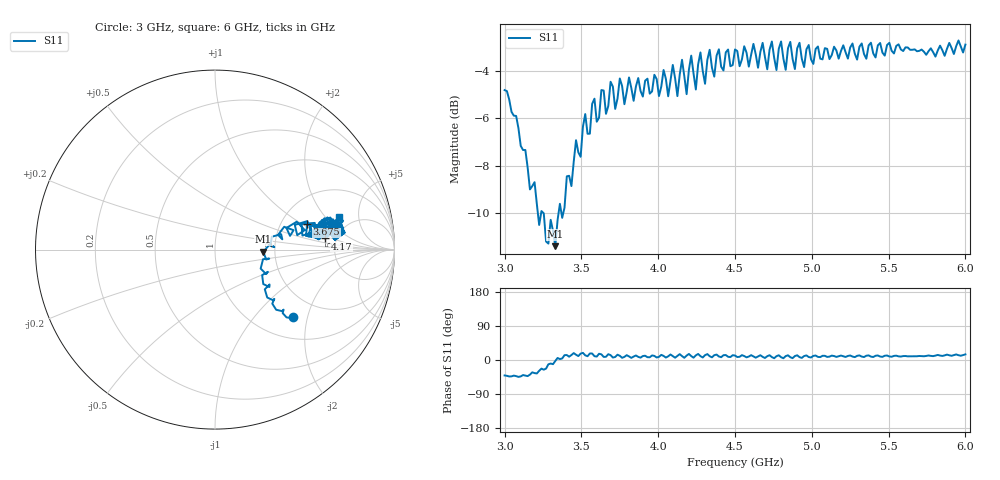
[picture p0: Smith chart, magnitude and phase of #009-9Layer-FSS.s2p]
!  05/08/2025  17:51:43
! Ref Plane: 0.000 mm
# MHZ S MA R  50
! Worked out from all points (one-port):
!   201 points, 3 GHz to 6 GHz, reference 50 ohm
!   lowest |S11| = -11.4 dB at 3.33 GHz (marker M1), VSWR 1.74, Z = 86.8 - j2.23 ohm
!   |S11| at or under -10 dB: 3.217 GHz to 3.238 GHz (21.13 MHz wide, 0.655 % of centre); 3.254 GHz to 3.351 GHz (96.73 MHz wide, 2.93 % of centre); 3.370074 GHz to 3.381806 GHz (11.73 MHz wide, 0.348 % of centre)
!   S11 on the Smith chart (normalised r, x): 3 GHz: 1.46, -1.63; 3.675 GHz: 2.79, +1.10; 4.17 GHz: 4.02, +0.81; 6 GHz: 3.80, +2.87
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3000  0.575 -40.7
3330  0.2695 -2.5
3375  0.3092 4.1
3525  0.5119 12.3
3675  0.5323 15.3
3750  0.6084 11.1
4095  0.6498 10.5
4125  0.5585 10.8
4170  0.615 5.8
4200  0.635 16.0
4230  0.6234 6.1
4260  0.6515 16.0
4290  0.6312 6.6
4320  0.6663 15.6
4350  0.6411 7.0
4500  0.7004 11.8
4695  0.6752 5.3
4725  0.6997 12.6
4755  0.6725 4.7
4785  0.7028 12.5
4815  0.6703 4.6
4845  0.7046 12.4
4875  0.6689 4.9
4905  0.7044 12.4
4935  0.6694 5.6
5250  0.7072 11.9
5625  0.7071 9.7
6000  0.7171 14.8
